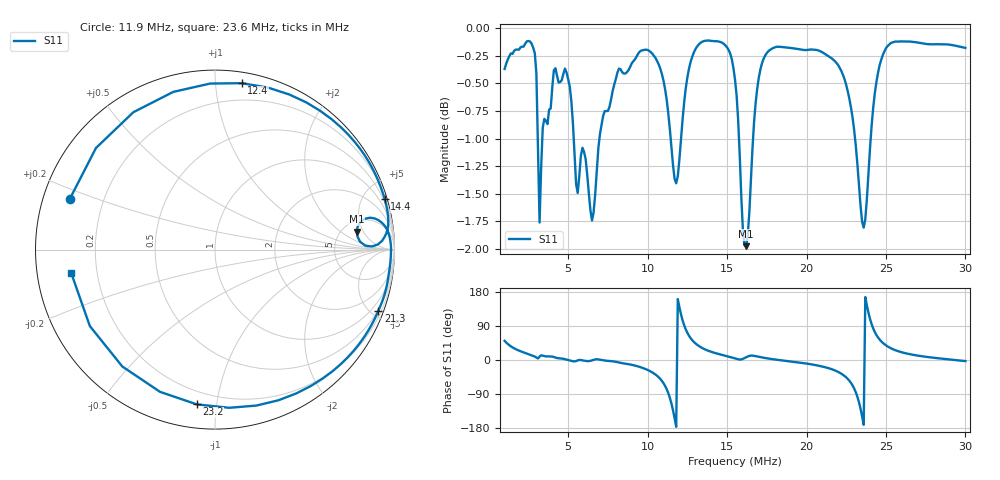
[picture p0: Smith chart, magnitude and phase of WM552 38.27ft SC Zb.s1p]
!Created via Zplots "Save as S1P" button
!Original data file:  $remote$.s1p
!Transmission line transform:  None
# MHZ S MA R 50
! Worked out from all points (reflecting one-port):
!   291 points, 1 MHz to 30 MHz, reference 50 ohm
!   lowest |S11| = -2.0 dB at 16.2 MHz (marker M1), VSWR 8.83, Z = 338 + j186 ohm
!   phase of S11 starts at 51 deg and turns -773 deg over the sweep
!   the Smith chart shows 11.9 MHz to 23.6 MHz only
!   S11 on the Smith chart (normalised r, x): 11.9 MHz: 0.08, +0.17; 12.4 MHz: 0.07, +1.17; 14.4 MHz: 0.33, +6.84; 21.3 MHz: 0.45, -5.50; 23.2 MHz: 0.13, -0.88; 23.6 MHz: 0.10, -0.08
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1  0.9583 50.6
2  0.9802 23.1
3.1  0.8833 4.0
4.7  0.9534 3.2
8.3  0.958 -7.6
10.4  0.9715 -35.5
10.9  0.9533 -55.2
11.3  0.915 -87.2
11.6  0.8667 -133.0
11.9  0.8569 160.8
12.1  0.8903 120.7
12.4  0.9391 80.8
13.1  0.9807 40.7
14.4  0.9865 16.6
15.5  0.9479 4.3
16.2  0.7966 7.3
19.2  0.9792 -4.9
21.3  0.972 -20.5
22.8  0.9205 -60.5
23.2  0.8683 -96.7
23.4  0.8312 -128.4
23.6  0.8121 -170.9
23.9  0.8598 124.7
24.1  0.9035 94.4
24.4  0.9454 66.1
24.9  0.976 41.8
26.4  0.9862 16.2
30  0.9797 -2.8
